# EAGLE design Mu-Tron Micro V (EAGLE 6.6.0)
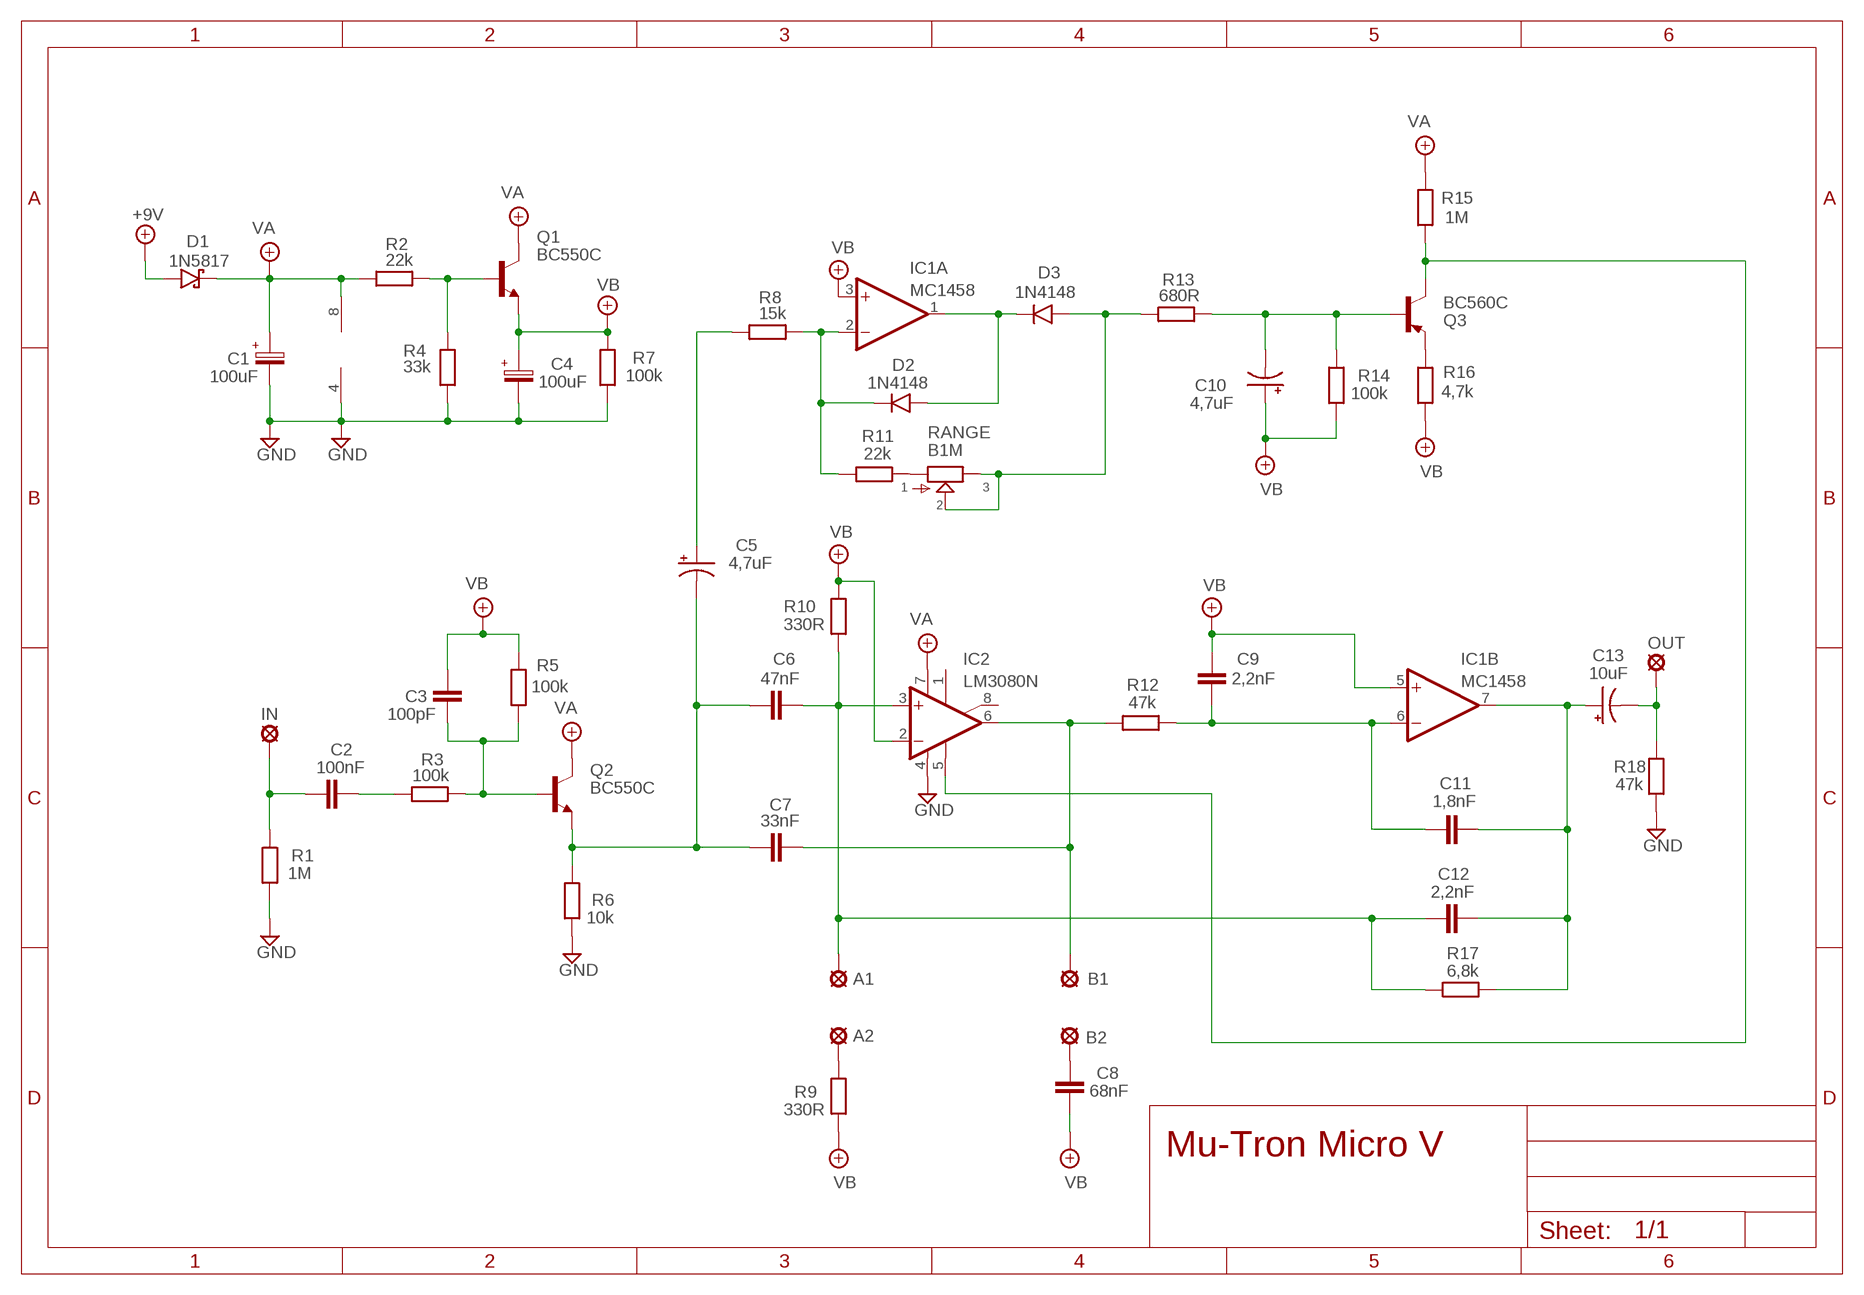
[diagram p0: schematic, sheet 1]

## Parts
+9V  +9V  +9V(T)1  [ROUND]
A1  MCS10B  [MCS10B]
A2  MCS10B  [MCS10B]
B1  MCS10B  [MCS10B]
B2  MCS10B  [MCS10B]
C1  100uF  063-EU  [063_025]
C2  100nF  100NF-220NF  [7,5MM]
C3  100pF  050X030_0251  [050X030_025]
C4  100uF  063-EU  [063_025]
C5  4,7uF  044A2  [044A_2]
C6  47nF  22NF-82NF"  [4,5MM]
C7  33nF  22NF-82NF"  [4,5MM]
C8  68nF  22NF-82NF"  [4,5MM]
C9  2,2nF  1NF-15NF  [3,5MM]
C10  4,7uF  044A2  [044A_2]
C11  1,8nF  1NF-15NF  [3,5MM]
C12  2,2nF  1NF-15NF  [3,5MM]
C13  10uF  044A2  [044A_2]
D1  1N5817  [DO41-3]
D2  1N4148  1N4148-3  [DO35-3]
D3  1N4148  1N4148-3  [DO35-3]
GND  GND  GND(T)1  [ROUND]
GND1  GND  GND(T)1  [ROUND]
IC1  MC1458  NE5532N  [DIL08]
IC2  LM3080N  [DIL08]
IN  MCS10B  [MCS10B]
OUT  MCS10B  [MCS10B]
Q1  BC550C  [TO92-EBC]
Q2  BC550C  [TO92-EBC]
Q3  BC560C  [TO92-EBC]
R1  1M  6MM-EU3  [R0207/3]
R2  22k  6MM-EU3  [R0207/3]
R3  100k  6MM-EU3  [R0207/3]
R4  33k  6MM-EU3  [R0207/3]
R5  100k  6MM-EU3  [R0207/3]
R6  10k  6MM-EU3  [R0207/3]
R7  100k  6MM-EU3  [R0207/3]
R8  15k  6MM-EU3  [R0207/3]
R9  330R  6MM-EU3  [R0207/3]
R10  330R  6MM-EU3  [R0207/3]
R11  22k  6MM-EU3  [R0207/3]
R12  47k  6MM-EU3  [R0207/3]
R13  680R  6MM-EU3  [R0207/3]
R14  100k  6MM-EU3  [R0207/3]
R15  1M  6MM-EU3  [R0207/3]
R16  4,7k  6MM-EU3  [R0207/3]
R17  6,8k  6MM-EU3  [R0207/3]
R18  47k  6MM-EU3  [R0207/3]
RANGE  B1M  POT-EU16MM  [16MM]

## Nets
+9V: +9V.1(+9V) D1.A
GND: C1.- C4.- GND1.1(GND) GND.1(GND) IC1.4(P:V-) IC2.4(V-) R1.1 R4.1 R6.1 R7.1 R18.1
N$1: C10.2(-) Q3.B R13.2 R14.2
N$2: Q1.B R2.2 R4.2
N$3: A1.MP C6.2 C12.1 IC2.3(+IN) R10.1 R17.1
N$4: IC2.5(OPT) Q3.C R15.1
N$5: Q3.E R16.2
N$6: C11.2 C12.2 C13.1(+) IC1.7(B:OUT) R17.2
N$7: C3.2 Q2.B R3.2 R5.1
N$8: C9.2 C11.1 IC1.6(B:-IN) R12.2
N$9: C2.P$2 R3.1
N$10: C2.P$1 IN.MP R1.2
N$11: C5.2(-) C6.1 C7.1 Q2.E R6.2
N$12: C13.2(-) OUT.MP R18.2
N$13: B2.MP C8.1
N$14: A2.MP R9.2
N$15: B1.MP C7.2 IC2.6(OUT) R12.1
N$16: D2.C IC1.2(A:-IN) R8.2 R11.1
N$17: C5.1(+) R8.1
N$19: D2.A D3.C IC1.1(A:OUT)
N$20: R11.2 RANGE.1
N$22: D3.A R13.1 RANGE.2 RANGE.3
VA: C1.+ D1.C IC1.8(P:V+) IC2.7(V+) Q1.C Q2.C R2.1 R15.2
VB: C3.1 C4.+ C8.2 C9.1 C10.1(+) IC1.3(A:+IN) IC1.5(B:+IN) IC2.2(-IN) Q1.E R5.2 R7.2 R9.1 R10.2 R14.1 R16.1
Unconnected: IC2.1(ON1) IC2.8(ON2)

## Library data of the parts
+9V = gm-supply:+9V(T): +9V Voltage Supply
A1 A2 B1 B2 IN OUT = Padit:MCS10B: SOLDER PAD
C1 C4 = Elektrolyytit:063-EU
C2 = Mylar Kondensaattorit:100NF-220NF: 100nF-220nF
C3 = Keraamiset kondensaattorit:050X030_025: 47 - 120pF
C5 C10 = Tantaalit:044A: .1 - 1.5µF
C6-C8 = Mylar Kondensaattorit:22NF-82NF: 22nF-82nF
C9 C11 C12 = Mylar Kondensaattorit:1NF-15NF: 1nF-15nF
C13 = gm-caps-tant:044A: .1 - 1.5µF
D1 = Diodit:1N5817
D2 D3 = Diodit:1N4148: Fast Switching Diode
GND GND1 = gm-supply:GND(T): Ground
IC1 = Operaatiovahvistimet:NE5532: AUDIO AMPLIFIER
IC2 = Operaatiovahvistimet:*3080: OP AMP
Q1 Q2 = transistor-npn:BC550*: NPN Transistor
Q3 = transistor-pnp:BC560*: PNP Transistror
R1-R18 = Vastukset:6MM-EU: 6mm Resistors (European schematic symbol)
RANGE = gm-pots:POT-EU

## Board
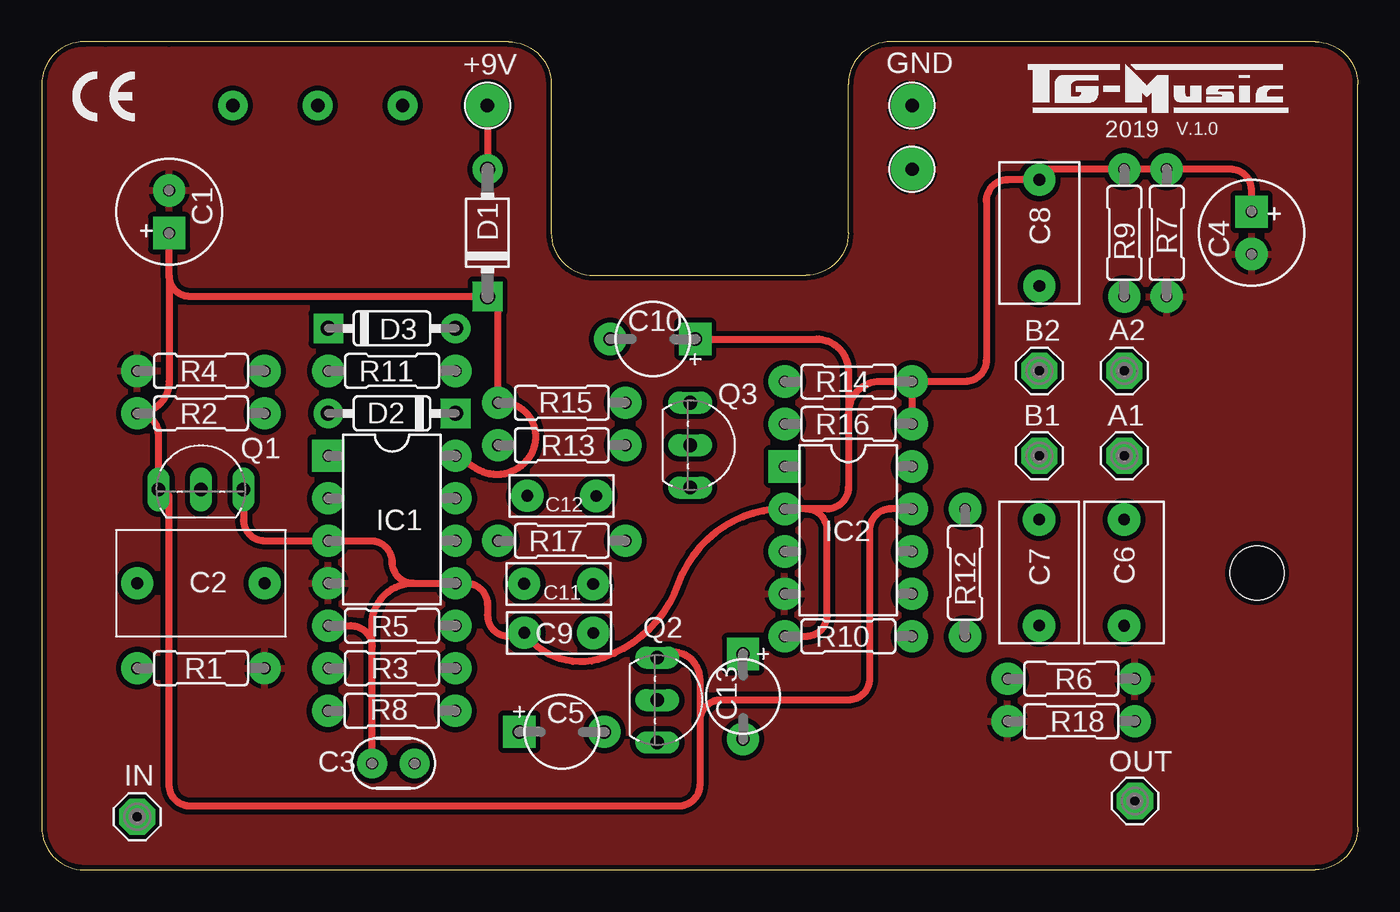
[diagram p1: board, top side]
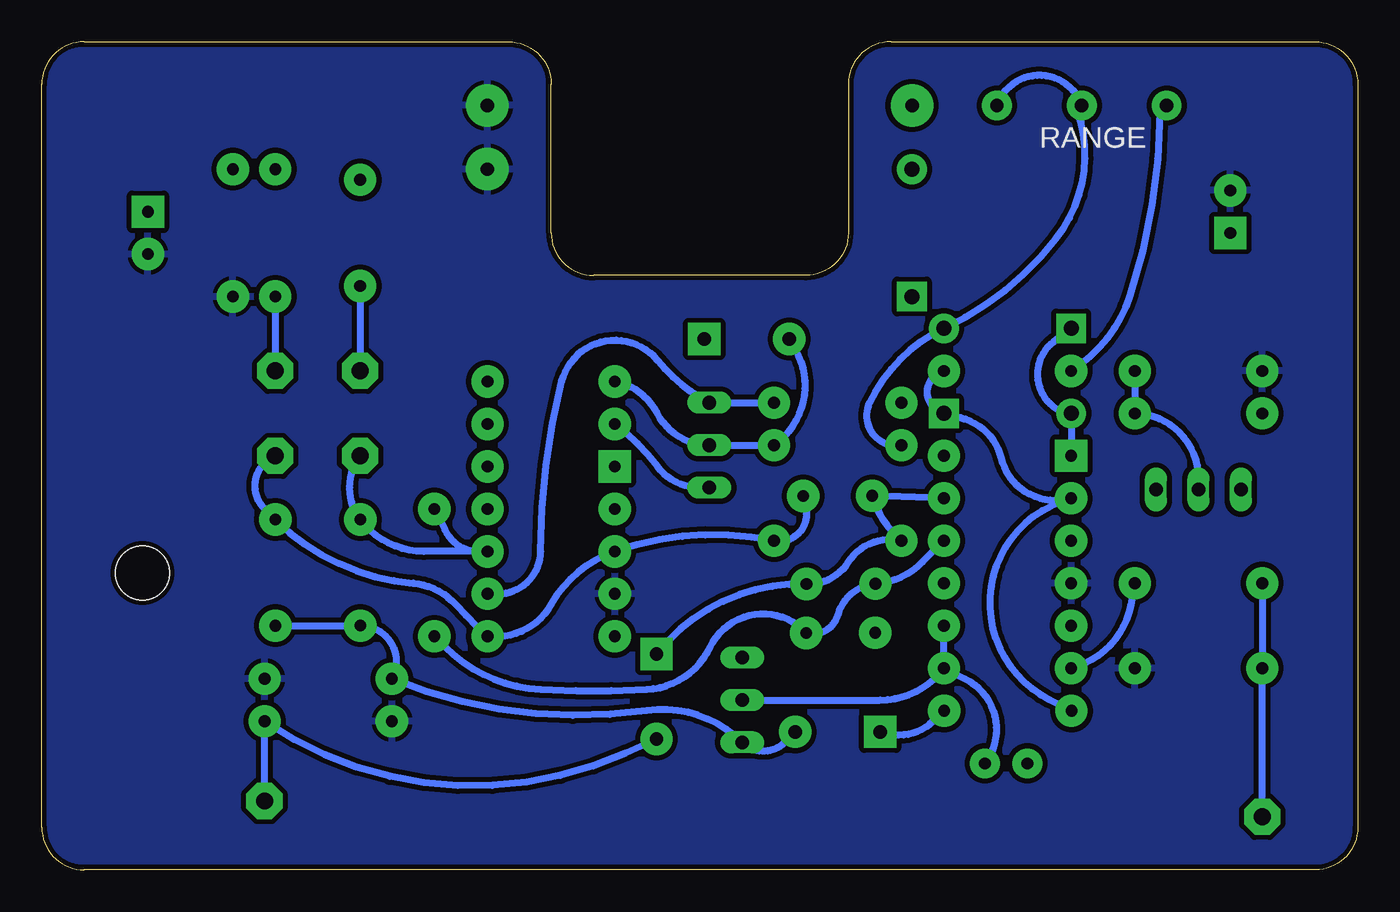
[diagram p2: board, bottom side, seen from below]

Size 78.74 x 49.53 mm. Coordinates in mm from the lower left corner, seen from the top.
Outline: 7.62,49.53 3.81,49.53
Outline: 78.74,2.54 78.74,46.99 arc90 76.2,49.53 50.8,49.53 arc90 48.26,46.99 48.26,38.1 arc-90 45.72,35.56 33.02,35.56 arc-90 30.48,38.1 30.48,46.99 arc90 27.94,49.53 2.54,49.53 arc90 0,46.99 0,2.54 arc90 2.54,0 76.2,0 arc90 78.74,2.54
Copper layers (1*16): Top 0.035mm / dielectric 1.5mm / Bottom 0.035mm
Design rules "ITEADstudio": minimum track width 10mil, minimum drill 12mil, track to track 12mil, track to pad 12mil, pad to pad 12mil, via to via 12mil, smd to smd 0mil, copper to edge 12mil, drill to drill 12mil, minimum pad ring 10mil, minimum via ring 6mil, stop-mask expansion 4mil, vias tented up to drill 100mil, thermal gap 10mil
Holes 3.2 mm at 72.71,17.76

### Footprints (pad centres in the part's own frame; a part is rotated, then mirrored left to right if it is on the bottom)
ROUND = drill 0.8 pad 2.54: 1 0,0
MCS10B = drill 1.016 pad 2.159 octagon: MP 0,0
063_025 = drill 0.7 pad 1.93 square: + -1.27,0 | drill 0.7 pad 1.93: - 1.27,0
7,5MM = drill 0.7 pad 1.93: P$1 -3.81,0; P$2 3.81,0
050X030_025 = drill 0.7 pad 1.778: 1 -1.27,0; 2 1.27,0
044A_2 = drill 0.8 pad 1.93 square: 1 -2.54,0 | drill 0.8 pad 1.93: 2 2.54,0
4,5MM = drill 0.7 pad 1.93: 1 -3.175,0; 2 3.175,0
3,5MM = drill 0.7 pad 1.93: 1 -1.905,0; 2 2.221,-0.016
DO41-3 = drill 0.9 pad 1.778: A 3.81,0 | drill 0.9 pad 1.778 square: C -3.81,0
DO35-3 = drill 0.9 pad 1.778: A 3.81,0 | drill 0.9 pad 1.778 square: C -3.81,0
DIL08 = drill 0.7 pad 1.93 square: 1 -3.81,-3.81 | drill 0.7 pad 1.93: 2 -1.27,-3.81; 3 1.27,-3.81; 4 3.81,-3.81; 5 3.81,3.81; 6 1.27,3.81; 7 -1.27,3.81; 8 -3.81,3.81
TO92-EBC = drill 0.813 long: B 0,-1.27; C -2.54,-1.27; E 2.54,-1.27
R0207/3 = drill 0.7 pad 1.93: 1 -3.81,0; 2 3.81,0
16MM = drill 0.8 pad 1.778: 1 5.08,0; 2 0,0; 3 -5.08,0

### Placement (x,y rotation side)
+9V  26.67,45.72 0 top
A1  64.77,24.77 0 top
A2  64.77,29.84 0 top
B1  59.69,24.77 0 top
B2  59.69,29.84 0 top
C1  7.62,39.37 90 top
C2  9.53,17.14 0 top
C3  21.04,6.37 0 top
C4  72.39,38.1 270 top
C5  31.11,8.26 0 top
C6  64.76,17.78 90 top
C7  59.68,17.78 90 top
C8  59.69,38.1 90 top
C9  30.78,14.18 0 top
C10  36.56,31.75 180 top
C11  30.76,17.11 0 top
C12  31.27,22.36 180 top
C13  41.96,10.37 270 top
D1  26.67,38.1 90 top
D2  20.95,27.3 180 top
D3  20.95,32.38 0 top
GND  52.07,45.72 0 top
GND1  52.07,41.91 0 top
IC1  20.95,20.95 270 top
IC2  48.26,20.32 270 top
IN  5.71,3.17 0 top
OUT  65.42,4.12 0 top
Q1  9.53,24.01 0 top
Q2  38.1,10.16 270 top
Q3  40.07,25.4 270 top
R1  9.53,12.06 180 top
R2  9.53,27.3 0 top
R3  20.95,12.06 0 top
R4  9.53,29.84 0 top
R5  20.95,14.61 180 top
R6  61.6,11.43 180 top
R7  67.31,38.1 90 top
R8  20.94,9.52 180 top
R9  64.77,38.1 270 top
R10  48.26,13.97 180 top
R11  20.95,29.84 180 top
R12  55.24,17.78 270 top
R13  31.11,25.4 0 top
R14  48.26,29.21 180 top
R15  31.11,27.94 180 top
R16  48.26,26.67 180 top
R17  31.11,19.68 180 top
R18  61.59,8.89 0 top
RANGE  16.51,45.72 0 bottom

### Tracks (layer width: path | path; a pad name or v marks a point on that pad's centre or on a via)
+9V
  Top 0.406: +9V.1 D1.A
GND
  pour Bottom: 0,1.91 0,46.99 arc-90 2.54,49.53 27.94,49.53 arc-90 30.48,46.99 30.48,38.1 arc90 33.02,35.56 45.72,35.56 arc90 48.26,38.1 48.26,46.99 arc-90 50.8,49.53 76.2,49.53 arc-90 78.74,46.99 78.74,1.91 arc-90 76.83,0 1.91,0 arc-90
  pour Top: 0,2.54 0,46.99 arc-90 2.54,49.53 27.94,49.53 arc-90 30.48,46.99 30.48,38.1 arc90 33.02,35.56 45.72,35.56 arc90 48.26,38.1 48.26,46.99 arc-90 50.8,49.53 76.2,49.53 arc-90 78.74,46.99 78.74,2.54 arc-90 76.2,0 2.54,0 arc-90
N$1
  Bottom 0.406: R14.2 arc52 41.91,27.3 arc-63 Q3.B R13.2 arc-85 33.66,31.11 C10.2
N$2
  Bottom 0.406: Q1.B 9.5,23.07 arc-92 R2.2 R4.2
N$3
  Bottom 0.406: C12.1 33.02,21.59 arc113 R17.1 arc-31 IC2.3 arc-41 48.26,15.88 arc68 R10.1 arc6 53.98,15.88 arc-43 56.52,17.14 arc40 C6.2 65.41,21.59 arc113 A1.MP
N$4
  Bottom 0.406: IC2.5 51.44,16.51 arc-90 48.9,19.05 arc14 47.62,29.21 arc126 41.91,30.48 arc-24 38.73,27.94 Q3.C R15.1
N$5
  Bottom 0.406: Q3.E 39.37,22.86 arc53 41.91,24.13 arc-16 R16.2
N$6
  Bottom 0.406: IC1.7 C12.2 28.78,21.7 arc-28 R17.2 arc-71 30.48,18.41 arc59 C11.2 arc-53 C13.1
N$7
  Bottom 0.406: R3.2 R5.1 | Q2.B 28.57,10.16 arc-53 R3.2 | R3.2 23.5,11.43 arc100 C3.2
N$8
  Bottom 0.406: IC1.6 26.04,18.41 arc40 C11.1 arc-70 31.11,15.24 arc90 C9.2 arc-112 38.73,13.34 arc62 42.55,10.79 arc6 48.9,10.79 arc42 54.61,13.34 R12.2
N$9
  Bottom 0.406: C2.P$2 13.58,15.85 arc65 R3.1
N$10
  Bottom 0.406: C2.P$1 R1.2 IN.MP
N$11
  Bottom 0.406: C5.2 34.29,7.62 arc90 Q2.E arc-53 42.55,9.53 arc31 R6.2 arc-118 C7.1 C6.1
N$12
  Bottom 0.406: OUT.MP R18.2 arc-59 43.81,6.99 C13.2
N$13
  Bottom 0.406: C8.1 B2.MP
N$14
  Bottom 0.406: R9.2 A2.MP
N$15
  Bottom 0.406: B1.MP arc-73 C7.2 arc-53 55.88,19.05 IC2.6 arc74 54.61,20.32 R12.1
N$16
  Bottom 0.406: R11.1 arc-151 D2.C 23.75,27.04 arc61 21.34,24.64 arc-92 IC1.2 arc-139 18.41,10.16 R8.2
N$17
  Bottom 0.406: R8.1 25.4,8.89 arc65 C5.1
N$19
  Bottom 0.406: D2.A 17.14,27.24 | 17.14,27.24 IC1.1 | D3.C 18.19,31.6 arc-133 17.14,27.24
N$20
  Bottom 0.406: R11.2 arc-40 13.63,34.37 arc-18 11.84,45.31 RANGE.1
N$22
  Bottom 0.406: RANGE.3 arc142 RANGE.2 16.76,45.47 arc57 18.05,37.76 arc26 D3.A arc-39 29.21,27.94 arc-125 R13.1
VA
  Top 0.406: 7.62,35.56 arc90 8.89,34.29 D1.C arc-90 27.3,33.66 R15.2 arc-116 29.45,25.24 arc-102 25.98,24.02 IC1.8 | 7.62,35.56 C1.+ | 7.62,35.56 7.62,29.21 arc-90 R2.1 arc-90 6.99,26.04 6.99,22.86 | Q1.C 6.99,22.86 | IC2.7 50.8,21.59 arc90 49.53,20.32 49.53,11.43 arc-90 48.26,10.16 40.64,10.16 arc90 39.37,8.89 | Q2.C arc-127 39.37,11.43 39.37,8.89 | 39.37,8.89 39.37,5.08 arc-90 38.1,3.81 8.89,3.81 arc-90 7.62,5.08 7.62,22.23 arc90 6.99,22.86
VB
  Top 0.406: Q1.E 12.06,20.95 arc90 13.34,19.68 IC1.3 19.68,19.68 arc-90 20.95,18.41 arc90 22.23,17.14 | 22.23,17.14 IC1.5 25.4,17.14 arc-90 26.67,15.88 26.67,15.24 arc90 27.94,13.97 28.66,13.97 arc90 C9.1 arc74 33.66,12.7 arc50 38.1,17.14 arc-70 IC2.2 45.72,21.59 | C3.1 19.77,13.34 | 19.77,13.34 19.77,14.69 arc-90 22.23,17.14 | R5.2 18.5,14.61 arc-90 19.77,13.34 | R14.1 R16.1 | 45.72,21.59 46.99,21.59 arc90 48.26,22.86 48.26,27.3 | R10.2 45.72,13.97 arc90 46.99,15.24 46.99,20.32 arc90 45.72,21.59 | C10.1 46.35,31.75 arc-90 48.26,29.84 48.26,27.3 | C4.+ 72.39,40.64 arc90 71.12,41.91 R7.2 R9.1 60.33,41.91 arc90 C8.2 57.78,41.27 arc90 56.52,40.01 56.52,30.48 arc-90 55.24,29.21 R14.1 | R14.1 50.16,29.21 arc90 48.26,27.3

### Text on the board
tNames: 2019 | V.1.0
